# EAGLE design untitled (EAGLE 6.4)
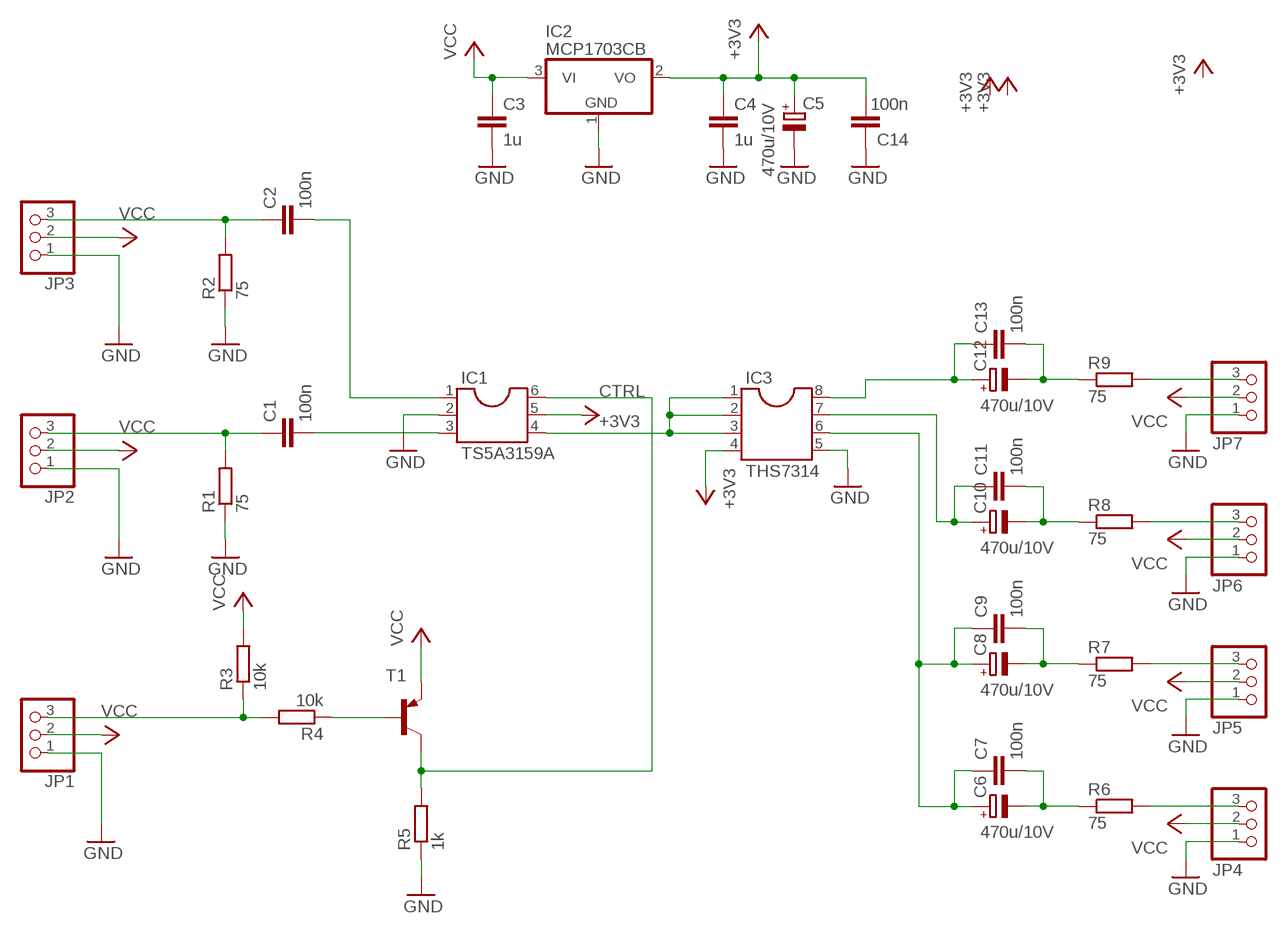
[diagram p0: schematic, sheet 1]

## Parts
C1  100n  C-EUC0805  [C0805]
C2  100n  C-EUC0805  [C0805]
C3  1u  C-EUC0805  [C0805]
C4  1u  C-EUC0805  [C0805]
C5  470u/10V  CPOL-EUD  [PANASONIC_D]
C6  470u/10V  CPOL-EUD  [PANASONIC_D]
C7  100n  C-EUC0805  [C0805]
C8  470u/10V  CPOL-EUD  [PANASONIC_D]
C9  100n  C-EUC0805  [C0805]
C10  470u/10V  CPOL-EUD  [PANASONIC_D]
C11  100n  C-EUC0805  [C0805]
C12  470u/10V  CPOL-EUD  [PANASONIC_D]
C13  100n  C-EUC0805  [C0805]
C14  100n  C-EUC0805  [C0805]
IC1  TS5A3159A  DIL6SOT  [SOT23-6L]
IC2  MCP1703CB  [SOT23]
IC3  THS7314  DIL8SMD  [SO08]
JP1  PINHD-1X3_KOLINOVO  [1X03]
JP2  PINHD-1X3_KOLINOVO  [1X03]
JP3  PINHD-1X3_KOLINOVO  [1X03]
JP4  PINHD-1X3_KOLINOVO  [1X03]
JP5  PINHD-1X3_KOLINOVO  [1X03]
JP6  PINHD-1X3_KOLINOVO  [1X03]
JP7  PINHD-1X3_KOLINOVO  [1X03]
R1  75  R-EU_R0805  [R0805]
R2  75  R-EU_R0805  [R0805]
R3  10k  R-EU_R0805  [R0805]
R4  10k  R-EU_R0805  [R0805]
R5  1k  R-EU_R0805  [R0805]
R6  75  R-EU_R0805  [R0805]
R7  75  R-EU_R0805  [R0805]
R8  75  R-EU_R0805  [R0805]
R9  75  R-EU_R0805  [R0805]
T1  BC807-16-PNP-SOT23-BEC  [SOT23-BEC]

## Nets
+3V3: C4.1 C5.+ C14.2 IC1.5 IC2.2(VO) IC3.4
CTRL: IC1.6 R5.2 T1.C
GND: C3.2 C4.2 C5.- C14.1 IC1.2 IC2.1(GND) IC3.5 JP1.1 JP2.1 JP3.1 JP4.1 JP5.1 JP6.1 JP7.1 R1.1 R2.1 R5.1
N$1: JP1.3 R3.1 R4.2
N$2: C2.1 JP3.3 R2.2
N$3: C1.1 JP2.3 R1.2
N$4: C12.+ C13.1 IC3.8
N$5: C12.- C13.2 R9.1
N$6: JP7.3 R9.2
N$7: C1.2 IC1.3
N$8: C2.2 IC1.1
N$9: C10.+ C11.1 IC3.7
N$10: C10.- C11.2 R8.1
N$11: JP6.3 R8.2
N$12: C6.+ C7.1 C8.+ C9.1 IC3.6
N$13: C8.- C9.2 R7.1
N$14: JP5.3 R7.2
N$15: IC1.4 IC3.1 IC3.2 IC3.3
N$16: C6.- C7.2 R6.1
N$17: JP4.3 R6.2
N$18: R4.1 T1.B
VCC: C3.1 IC2.3(VI) JP1.2 JP2.2 JP3.2 JP4.2 JP5.2 JP6.2 JP7.2 R3.2 T1.E

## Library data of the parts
C1-C4 C7 C9 C11 C13 C14 = rcl:C-EU: CAPACITOR, European symbol
C5 C6 C8 C10 C12 = rcl:CPOL-EU: POLARIZED CAPACITOR, European symbol
IC1 = ic-package:DIL6: Dual In Line / Socket
IC2 = linear:MCP1703: 250 mA, 16V, Low Quiescent Current LDO Regulator Source: http://ww1.microchip.com/downloads/en/DeviceDoc/22049b.pdf
IC3 = ic-package:DIL8: Dual In Line / Socket
JP1-JP7 = PINHEAD_RC:PINHD-1X3_KOLINOVO: KOLINOVO PIN HEADER
R1-R9 = rcl:R-EU_: RESISTOR, European symbol
T1 = transistor-neu-to92:*-PNP-: PNP Transistror

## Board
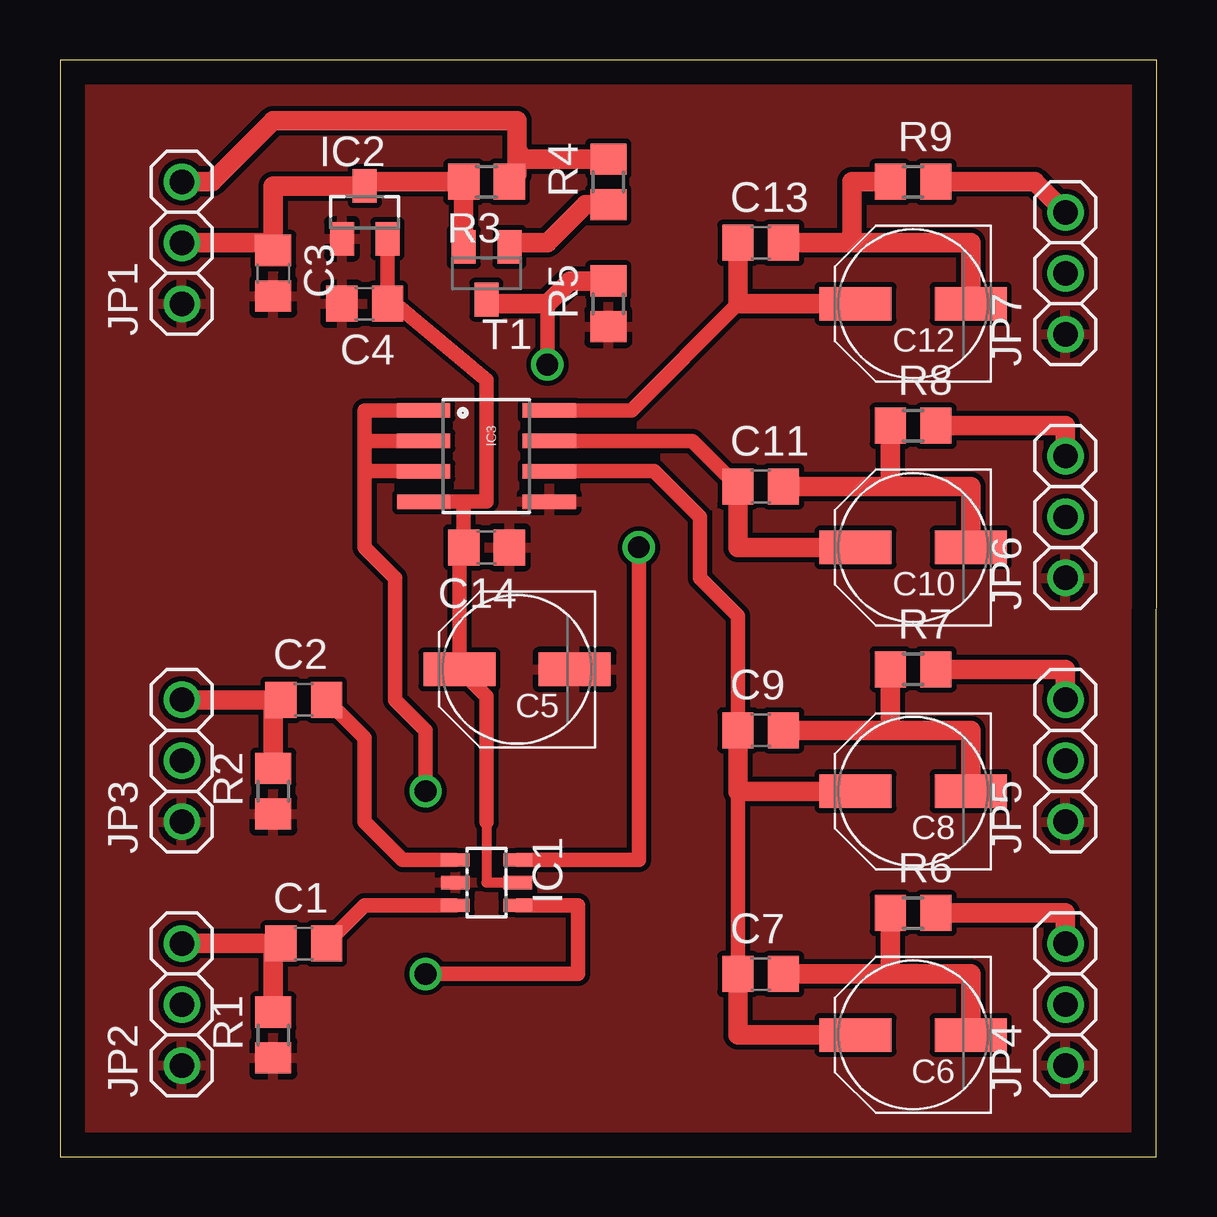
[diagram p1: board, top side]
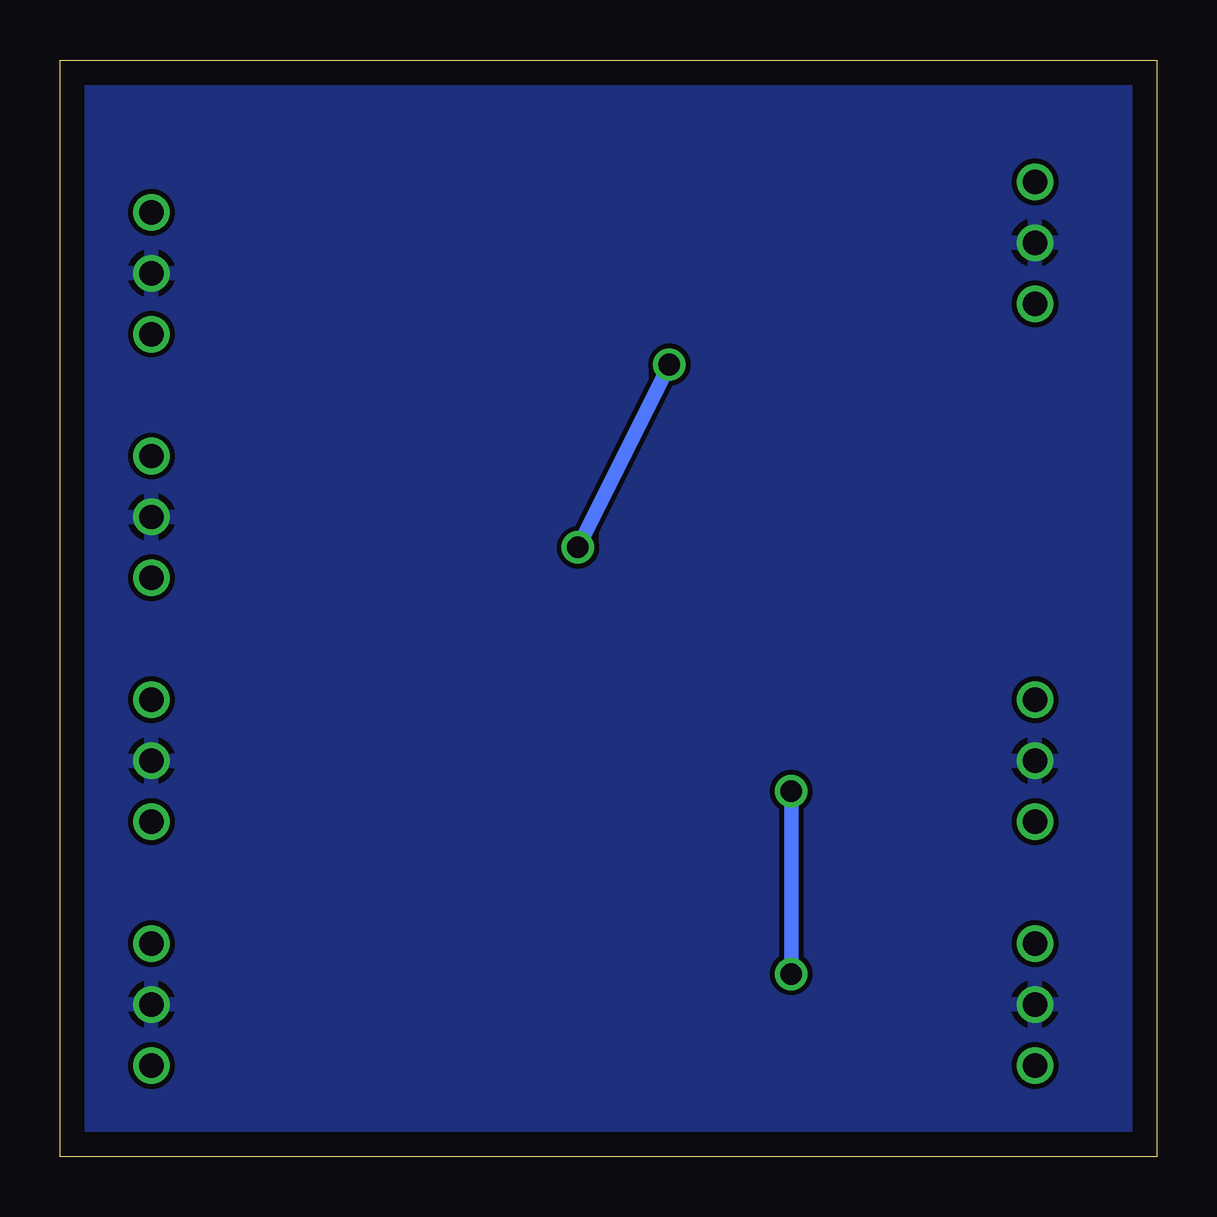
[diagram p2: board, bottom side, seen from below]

Size 45.72 x 45.72 mm. Coordinates in mm from the lower left corner, seen from the top.
Outline: 0,0 45.7,0 45.72,45.72 0,45.72 0,0
Copper layers (1*16): Top 0.035mm / dielectric 1.5mm / Bottom 0.035mm
Design rules "default": minimum track width 10mil, minimum drill 24mil, track to track 8mil, track to pad 8mil, pad to pad 8mil, via to via 8mil, smd to smd 8mil, copper to edge 40mil, drill to drill 8mil, minimum pad ring 10mil, minimum via ring 8mil, stop-mask expansion 4mil, vias tented up to drill 0mil, thermal gap 10mil

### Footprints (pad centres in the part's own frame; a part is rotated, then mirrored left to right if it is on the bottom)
C0805 = smd 1.3 x 1.5: 1 -0.95,0; 2 0.95,0
PANASONIC_D = smd 3 x 1.4: + 2.4,0; - -2.4,0
SOT23-6L = smd 0.55 x 1.2: 1 -0.95,-1.3; 2 0,-1.3; 3 0.95,-1.3; 4 0.95,1.3; 5 0,1.3; 6 -0.95,1.3
SOT23 = smd 1 x 1.4: 1 -0.95,-1.1; 2 0.95,-1.1; 3 0,1.1
SO08 = smd 0.61 x 2.21: 1 -1.905,-2.616; 2 -0.635,-2.616; 3 0.635,-2.616; 4 1.905,-2.616; 5 1.905,2.616; 6 0.635,2.616; 7 -0.635,2.616; 8 -1.905,2.616
1X03 = drill 1.016: 1 -2.54,0; 2 0,0; 3 2.54,0
R0805 = smd 1.3 x 1.5: 1 -0.95,0; 2 0.95,0
SOT23-BEC = smd 1 x 1.4: B -0.95,-1.1; C 0,1.1; E 0.95,-1.1

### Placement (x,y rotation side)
C1  10.16,8.89 0 top
C2  10.16,19.05 0 top
C3  8.89,36.83 270 top
C4  12.7,35.56 180 top
C5  19.05,20.32 180 top
C6  35.56,5.08 180 top
C7  29.21,7.62 0 top
C8  35.56,15.24 180 top
C9  29.21,17.78 0 top
C10  35.56,25.4 180 top
C11  29.21,27.94 0 top
C12  35.56,35.56 180 top
C13  29.21,38.1 0 top
C14  17.78,25.4 180 top
IC1  17.78,11.43 270 top
IC2  12.7,39.37 0 top
IC3  17.78,29.21 270 top
JP1  5.08,38.1 90 top
JP2  5.08,6.35 90 top
JP3  5.08,16.51 90 top
JP4  41.91,6.35 90 top
JP5  41.91,16.51 90 top
JP6  41.91,26.67 90 top
JP7  41.91,36.83 90 top
R1  8.89,5.08 90 top
R2  8.89,15.24 90 top
R3  17.78,40.64 180 top
R4  22.86,40.64 90 top
R5  22.86,35.56 90 top
R6  35.56,10.16 0 top
R7  35.56,20.32 0 top
R8  35.56,30.48 0 top
R9  35.56,40.64 0 top
T1  17.78,36.83 180 top

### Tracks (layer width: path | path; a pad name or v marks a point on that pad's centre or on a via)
+3V3
  Top 0.406: 17.78,13.97 17.78,11.43 IC1.5
  Top 0.61: IC3.4 16.83,27.3 | 16.83,27.3 C14.2 16.65,25.4 C5.+ 17.78,19.19 17.78,13.97 | IC2.2 C4.1 13.97,35.56 17.78,32.38 17.78,27.3 16.83,27.3
CTRL  (via drill 0.9)
  Top 0.61: IC1.6 24.13,12.38 v24.13,25.4 | v20.32,33.02 20.32,35.56
  Top 0.813: R5.2 21.27,36.51 20.32,35.56 17.95,35.56 T1.C
  Bottom 0.61: v24.13,25.4 v20.32,33.02
GND
  pour Top: 0,0 45.72,0 45.72,45.72 0,45.72
N$1
  Top 0.813: JP1.3 6.35,40.64 8.89,43.18 19.05,43.18 19.05,41.91 | 19.05,41.91 19.05,40.96 R3.1 | R4.2 19.37,41.59 19.05,41.91
N$2
  Top 0.813: JP3.3 C2.1 8.89,18.73 R2.2
N$3
  Top 0.813: R1.2 8.89,8.57 C1.1 JP2.3
N$4
  Top 0.61: IC3.8 23.82,31.11 28.26,35.56
  Top 0.813: C13.1 28.26,35.56 C12.+
N$5
  Top 0.813: R9.1 33.02,40.64 33.02,38.1 | 33.02,38.1 C13.2 | C12.- 37.96,38.1 33.02,38.1
N$6
  Top 0.813: JP7.3 40.64,40.64 R9.2
N$7
  Top 0.61: C1.2 12.7,10.48 IC1.3
N$8
  Top 0.61: C2.2 12.7,17.46 12.7,13.97 14.29,12.38 IC1.1
N$9
  Top 0.61: IC3.7 26.36,29.84 C11.1
  Top 0.813: C11.1 28.26,25.4 C10.+
N$10
  Top 0.813: R8.1 34.61,27.94 | 34.61,27.94 C11.2 | C10.- 37.96,27.94 34.61,27.94
N$11
  Top 0.813: JP6.3 41.91,30.48 R8.2
N$12
  Top 0.61: IC3.6 24.77,28.57 26.67,26.67 26.67,24.13 28.26,22.54 C9.1 | C7.1 28.26,15.24
  Top 0.813: C9.1 28.26,15.24 C8.+ | C7.1 28.26,5.08 C6.+
N$13
  Top 0.813: R7.1 34.61,17.78 | 34.61,17.78 C9.2 | C8.- 37.96,17.78 34.61,17.78
N$14
  Top 0.813: JP5.3 41.91,20.32 R7.2
N$15  (via drill 0.9)
  Top 0.61: IC3.1 12.7,31.11 12.7,29.84 | IC3.2 12.7,29.84 | IC3.3 12.7,28.57 | 12.7,28.57 12.7,29.84 | IC1.4 21.59,10.48 21.59,7.62 v15.24,7.62 | v15.24,15.24 15.24,17.78 13.97,19.05 13.97,24.13 12.7,25.4 12.7,28.57
  Bottom 0.61: v15.24,7.62 v15.24,15.24
N$16
  Top 0.813: R6.1 34.61,7.62 | 34.61,7.62 C7.2 | C6.- 37.96,7.62 34.61,7.62
N$17
  Top 0.813: JP4.3 41.91,10.16 R6.2
N$18
  Top 0.813: R4.1 21.91,39.69 20.32,38.1 18.9,38.1 T1.B
VCC
  Top 0.813: JP1.2 8.57,38.1 arc-90 C3.1 8.89,40.47 IC2.3 12.87,40.64 R3.2 T1.E
  pour Bottom: 0,0 45.72,0 45.72,45.72 0,45.72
